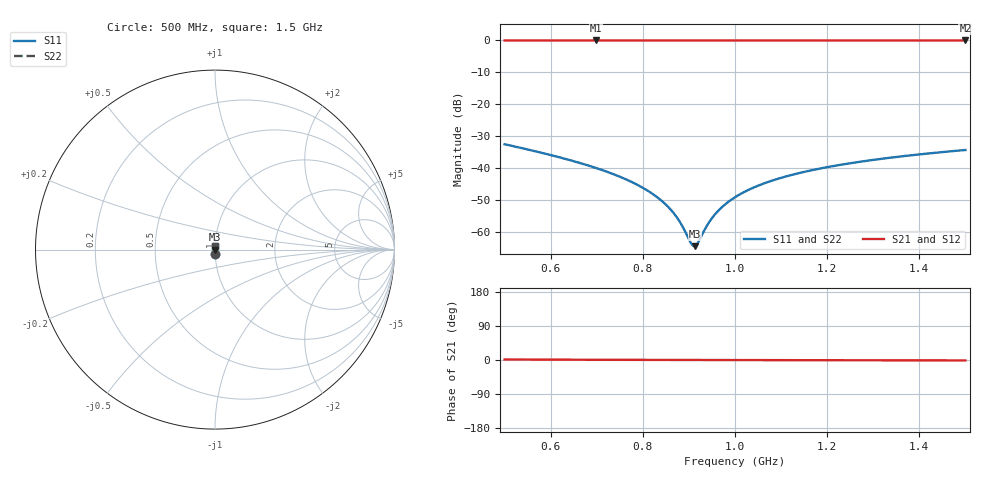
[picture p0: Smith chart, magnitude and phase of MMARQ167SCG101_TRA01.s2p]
! MMARQ167SCG101_TRA01  S-PARAMETER MODEL  ( General Type )
! Model Generated by TAIYO YUDEN Corporation (http://www.ty-top.com)
! Version 1.0
! TAIYO YUDEN Control No. 150609
! Copyright(c) 2015 TAIYO YUDEN CO.,LTD. All Rights Reserved.
! Product Description (link to TY-COMPAS)
! https://ds.yuden.co.jp/TYCOMPAS/or/detail?pn=MMARQ167SCG101JTRA01&u=M
! Products Name : Multilayer Ceramic Capacitors
! Characteristics :
!  Capacitance : 100 pF , Rated Voltage : 250V , TCC : CG / C0G
!  Case Size : 1.6 x 0.8 / 0.063 x 0.031 [mm/inch] , Thickness : 0.7 / 0.028 [mm/inch]
!  (Conditions: Temperature = 25 degC , DC Bias Current/Voltage = 0A / 0V)
! External Node Assignments :
!  1  o---| |---o  2
! GND o---------o GND
! Frequency Range : 500MHz  -  1.5GHz  [ 401 STEP ]
# MHz S RI R 50
! Freq[MHz].  S11 Real  S11 Imag  S21 Real  S21 Imag  S12 Real  S12 Imag  S22 Real  S22 Imag
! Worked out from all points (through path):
!   401 points, 500 MHz to 1.5 GHz, reference 50 ohm
!   highest |S21| = 0.00 dB at 697.5 MHz (marker M1); lowest = 0.0 dB at 1.5 GHz (marker M2)
!   lowest |S11| = -64.5 dB at 912.5 MHz (marker M3), VSWR 1.00, Z = 50.1 + j0.0018 ohm
!   |S11| at or under -10 dB: start of sweep to end of sweep
!   |S22| runs from -64.5 to -32.6 dB; largest |S21 - S12| = 0
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500  0.000926 -0.0235  0.9991 0.0235  0.9991 0.0235  0.000926 -0.0235
667.5  0.000557 -0.0117  0.9994 0.0117  0.9994 0.0117  0.000557 -0.0117
697.5  0.000536 -0.01  0.9995 0.01  0.9995 0.01  0.000536 -0.01
777.5  0.000521 -0.00592  0.9995 0.00592  0.9995 0.00592  0.000521 -0.00592
810  0.000528 -0.00439  0.9995 0.00439  0.9995 0.00439  0.000528 -0.00439
835  0.000539 -0.00326  0.9995 0.00326  0.9995 0.00326  0.000539 -0.00326
855  0.00055 -0.00239  0.9995 0.00239  0.9995 0.00239  0.00055 -0.00239
870  0.000559 -0.00174  0.9994 0.00174  0.9994 0.00174  0.000559 -0.00174
885  0.00057 -0.00111  0.9994 0.00111  0.9994 0.00111  0.00057 -0.00111
905  0.000586 -0.000286  0.9994 0.000286  0.9994 0.000286  0.000586 -0.000286
912.5  0.000592 1.8e-05  0.9994 -1.8e-05  0.9994 -1.8e-05  0.000592 1.8e-05
920  0.000599 0.00032  0.9994 -0.00032  0.9994 -0.00032  0.000599 0.00032
940  0.000618 0.00111  0.9994 -0.00111  0.9994 -0.00111  0.000618 0.00111
955  0.000634 0.0017  0.9994 -0.0017  0.9994 -0.0017  0.000634 0.0017
975  0.000656 0.00246  0.9993 -0.00246  0.9993 -0.00246  0.000656 0.00246
1000  0.000686 0.0034  0.9993 -0.0034  0.9993 -0.0034  0.000686 0.0034
1032.5  0.000729 0.00458  0.9993 -0.00458  0.9993 -0.00458  0.000729 0.00458
1070  0.000782 0.00591  0.9992 -0.00591  0.9992 -0.00591  0.000782 0.00591
1167.5  0.000943 0.00919  0.9991 -0.00919  0.9991 -0.00919  0.000943 0.00919
1245  0.00109 0.0116  0.9989 -0.0116  0.9989 -0.0116  0.00109 0.0116
1335  0.00128 0.0144  0.9987 -0.0144  0.9987 -0.0144  0.00128 0.0144
1500  0.00168 0.0191  0.9983 -0.0191  0.9983 -0.0191  0.00168 0.0191
